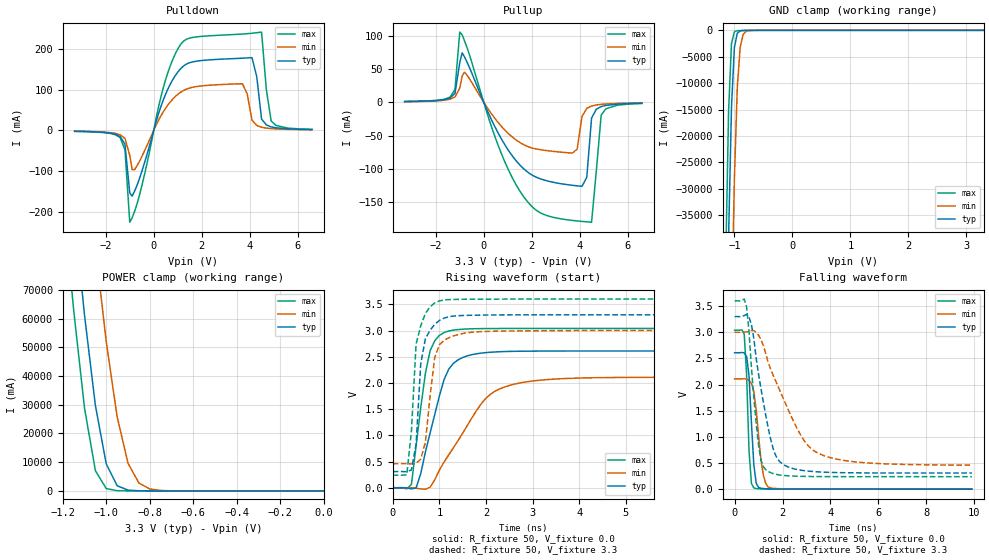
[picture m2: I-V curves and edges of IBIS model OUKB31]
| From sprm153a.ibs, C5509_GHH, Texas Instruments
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| Pin_model   OUKB31
[Model]   OUKB31
 Model_type   3-state
 Polarity   Non-Inverting
 Enable   Active-Low
 Vmeas =  1.5
|Variable   typ   min   max
 C_comp   2.629pF   2.529pF   2.786pF
[Temperature Range]   25   125   -40
[Voltage Range]   3.3   3   3.6
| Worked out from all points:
|   slope of the pulldown table from 0 to 0.495 V, typ, clamps not added: 5.59 ohm
|   slope of the pullup table from 0 to 0.495 V, typ, clamps not added: 12.7 ohm
|   GND clamp passes 1 mA (typ) near -0.58 V on its own axis
|   POWER clamp passes 1 mA (typ) near -0.64 V on its own axis
|   rising waveform, R_fixture 50, V_fixture 0.0: 20-80 % time 452ps typ, 922ps min, 283ps max; typ from 0 V to 2.61 V
|   rising waveform, R_fixture 50, V_fixture 3.3: 20-80 % time 165ps typ, 192ps min, 174ps max; typ from 0.308 V to 3.3 V
|   falling waveform, R_fixture 50, V_fixture 0.0: 20-80 % time 184ps typ, 295ps min, 152ps max; typ from 2.61 V to 0 V
|   falling waveform, R_fixture 50, V_fixture 3.3: 20-80 % time 684ps typ, 1.49ns min, 369ps max; typ from 3.3 V to 0.308 V
[GND Clamp]
|Voltage   I(typ)   I(min)   I(max)
-3.3V     -2.136kA   -2.179kA   -2.116kA
-1.15V    -73.18A    -126.6A    -44.15A
-1.1V     -39.22A    -88.81A    -15.39A
-1.05V    -14.62A    -55.16A    -2.49A
-1V       -3.284A    -28.2A     -287.3mA
-950mV    -553.9mA   -10.89A    -70.37mA
-900mV    -106.4mA   -3.191A    -41.81mA
-850mV    -34.73mA   -810.3mA   -29.9mA
-800mV    -18.69mA   -202.8mA   -20.42mA
-600mV    -1.349mA   -2.989mA   -882.6uA
3.3V      215.8pA    2.558nA    183pA
[POWER Clamp]
|Voltage   I(typ)   I(min)   I(max)
-3.3V     2.17kA     2.223kA    2.142kA
-1.2V     139.9A     204.8A     103.2A
-1.15V    98.84A     162.7A     63.07A
-1.1V     61.17A     122.4A     28.82A
-1.05V    29.72A     84.94A     7.071A
-1V       9.377A     51.87A     811.7mA
-950mV    1.804A     25.81A     78.35mA
-900mV    278.3mA    9.635A     13.2mA
-850mV    43.85mA    2.746A     6.214mA
-800mV    9.014mA    681.5mA    4.323mA
-750mV    3.227mA    163mA      3.037mA
0V        0A         0A         0A
[Pulldown]
|Voltage   I(typ)   I(min)   I(max)
-3.3V     -2.2mA     -1.9mA     -2.4mA
-1.4V     -15.07mA   -10.71mA   -17.62mA
-1.2V     -33.87mA   -19.73mA   -47.74mA
-1V       -153.2mA   -61.06mA   -225mA
-800mV    -149.2mA   -96.14mA   -198.8mA
400mV     74.55mA    45.59mA    104.5mA
1.1V      149.7mA    92.53mA    208.7mA
3.7V      177mA      114.4mA    236.2mA
4.1V      178.4mA    25.21mA    238.1mA
4.5V      27.87mA    7.75mA     241mA
4.9V      8.67mA     4.45mA     23.18mA
6.6V      2.1mA      1.6mA      2.6mA
[Pullup]
|Voltage   I(typ)   I(min)   I(max)
-3.3V     1.1mA      900uA      1.1mA
-1.4V     6.47mA     4.63mA     7.89mA
-1.2V     13.26mA    7.95mA     19.14mA
-1V       59.39mA    21.19mA    105.4mA
900mV     -64.96mA   -42.43mA   -91.14mA
2.25V     -113.5mA   -70.61mA   -163.7mA
3.7V      -124.8mA   -76.4mA    -177.6mA
4.1V      -126.4mA   -21.53mA   -179.1mA
4.3V      -112.9mA   -9.24mA    -179.7mA
4.5V      -23.75mA   -5.67mA    -180.2mA
4.9V      -6.54mA    -3.14mA    -19.41mA
6.6V      -1.5mA     -1.1mA     -1.9mA
[Ramp]
|Variable   typ   min   max
 dV/dt_r   1.56V/0.450ns   1.27V/0.930ns   1.80V/0.270ns
 dV/dt_f   1.78V/0.680ns   1.53V/1.490ns   2.03V/0.370ns
 R_load =  50
[Rising Waveform]
 R_fixture =   50
 V_fixture =   0.0
 V_fixture_min =  0.0
 V_fixture_max =  0.0
|Time   V(typ)   V(min)   V(max)
0s        1.927nV    21.89uV    9.892nV
400ps     -22.25mV   -565.5uV   62.27mV
500ps     -4.453mV   -9.722mV   793.9mV
700ps     681.1mV    -27.19mV   2.183V
800ps     1.043V     8.309mV    2.611V
1.1ns     2.061V     490mV      2.962V
1.4ns     2.44V      898.3mV    3.018V
2ns       2.579V     1.709V     3.037V
2.7ns     2.604V     1.994V     3.039V
9.9ns     2.609V     2.108V     3.039V
[Rising Waveform]
 R_fixture =   50
 V_fixture =   3.3
 V_fixture_min =  3
 V_fixture_max =  3.6
|Time   V(typ)   V(min)   V(max)
0s        308.5mV    459mV      239.2mV
300ps     304.5mV    458.9mV    245.9mV
400ps     340.7mV    455mV      1.077V
500ps     827mV      465.9mV    2.74V
600ps     2.366V     544.9mV    3.089V
700ps     2.842V     870.1mV    3.326V
900ps     3.118V     2.485V     3.525V
1ns       3.192V     2.728V     3.565V
2ns       3.295V     2.982V     3.599V
9.9ns     3.3V       3V         3.6V
[Falling Waveform]
 R_fixture =   50
 V_fixture =   0.0
 V_fixture_min =  0.0
 V_fixture_max =  0.0
|Time   V(typ)   V(min)   V(max)
0s        2.609V     2.108V     3.039V
400ps     2.606V     2.112V     2.964V
500ps     2.535V     2.107V     2.182V
600ps     2.166V     2.083V     736.9mV
700ps     1.272V     2.023V     110mV
800ps     467.3mV    1.868V     24.59mV
900ps     114.5mV    1.513V     10.77mV
1.1ns     17.86mV    558.3mV    5.301mV
1.4ns     6.418mV    41.28mV    3.077mV
9.9ns     -431nV     21.57uV    22.47nV
[Falling Waveform]
 R_fixture =   50
 V_fixture =   3.3
 V_fixture_min =  3
 V_fixture_max =  3.6
|Time   V(typ)   V(min)   V(max)
0s        3.3V       3V         3.6V
500ps     3.341V     3.008V     3.479V
700ps     3.148V     3.031V     2.328V
1ns       2.191V     2.942V     834.7mV
1.3ns     1.409V     2.585V     371.2mV
1.6ns     786mV      2.186V     298.9mV
1.9ns     518.9mV    1.871V     270.4mV
2.8ns     360.4mV    999.5mV    245.2mV
3.4ns     333.1mV    708.9mV    241.1mV
9.9ns     308.5mV    459mV      239.2mV
